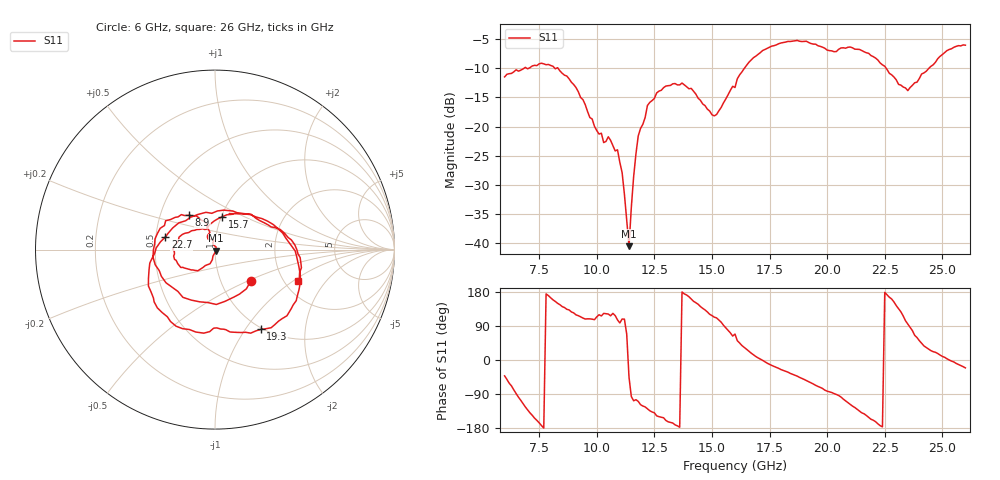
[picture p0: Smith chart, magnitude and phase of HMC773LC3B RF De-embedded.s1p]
! Hittite Microwave Corporation
! 20 Alpha Road
! Chelmsford, MA 01824
! http://www.hittite.com
! Tel: 978-250-3343
! Fax: 978-250-3373
! Device:  HMC773LC3B
! Description: GaAS MMIC Fundamental Mixer
! Frequency:  6-  26 GHz Mixer
! Package:  LC3B - 3x3 mm QFN Ceramic High frequency SMT Package: 12 pin
! Ports
!  Pin  2  = LO
!  Pin  5  = IF
!  pin  8  = RF
! Data:  The device was measured on evaluation board 125040-1.
!  The evaluation circuit board was modeled and simulated.  This was use
!  to removed the evaluation board circuit from the measured data.
!  The reference plane is the center of the package pin.
! Misc:
! Date Measured:  09-10-2009
! Date:  09-10-2009
! Note:
!  Hittite supplies this data as a sample of measured data at the package pin for
!  for this package product.  Your particular data for this product may vary.
!  Data was taken at 25 degrees C.
!  Hittite reserves the right to change this data at anytime.
# MHz S MA R 50
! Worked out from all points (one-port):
!   201 points, 6 GHz to 26 GHz, reference 50 ohm
!   lowest |S11| = -40.5 dB at 11.4 GHz (marker M1), VSWR 1.02, Z = 50.7 - j0.687 ohm
!   |S11| at or under -10 dB: start of sweep to 6.856 GHz; 8.311 GHz to 16.41 GHz (8.102 GHz wide, 65.5 % of centre); 22.56 GHz to 24.43 GHz (1.87 GHz wide, 7.96 % of centre)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
!   S11 on the Smith chart (normalised r, x): 6 GHz: 1.38, -0.53; 8.9 GHz: 0.70, +0.28; 15.7 GHz: 1.01, +0.38; 19.3 GHz: 0.98, -1.18; 22.7 GHz: 0.56, +0.09; 26 GHz: 2.37, -1.11
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6000  0.2658 -41.9
6500  0.3057 -88.6
7500  0.3437 -165.8
8500  0.2853 141.0
8900  0.2391 126.8
10300  0.07296 123.0
10500  0.08178 121.3
10900  0.06322 105.9
11000  0.04957 97.8
11100  0.04046 108.1
11400  0.009483 -45.6
11600  0.03713 -107.5
11800  0.08317 -109.2
12200  0.1515 -128.9
12600  0.1938 -147.4
13500  0.2271 -173.7
15100  0.1233 113.1
15700  0.187 77.6
16000  0.2157 68.4
17200  0.4467 -1.0
18500  0.5372 -37.7
19300  0.5124 -60.1
21000  0.4787 -116.9
21800  0.4229 -151.3
22700  0.2849 165.5
23500  0.2029 95.0
24900  0.3983 13.1
26000  0.4964 -20.9
